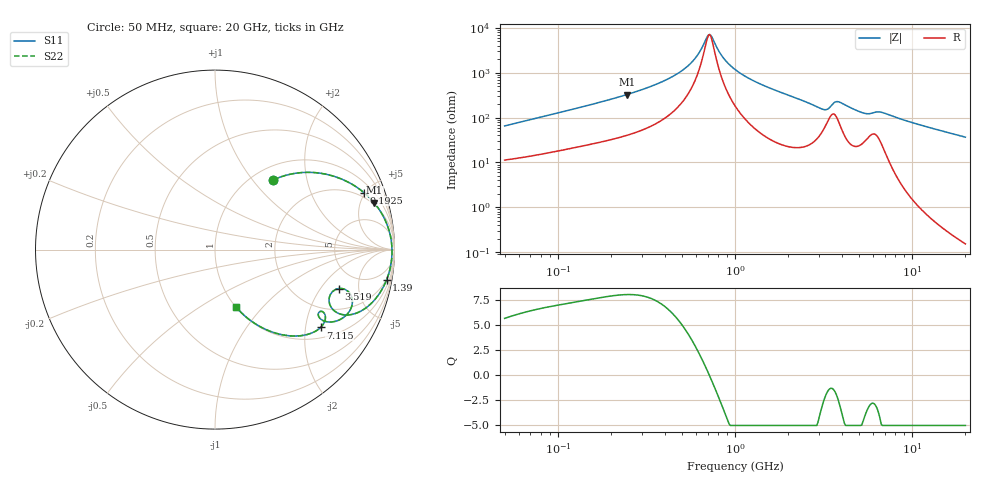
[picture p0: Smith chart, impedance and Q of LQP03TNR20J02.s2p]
!Murata Part Number: LQP03TNR20J02
!These Parameters are Measured in Series Mode Connection
!  o--[Z]--o
!Port1  Port2
!  o-------o
!Freq. Start=50[MHz] Stop=20[GHz], 401[Steps]
# Hz S RI R 50
!Freq.(Hz) S11(Real) S11(Imag) S21(Real) S21(Imag) S12(Real) S12(Imag) S22(Real) S22(Imag)
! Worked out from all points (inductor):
!   401 points, 50 MHz to 20 GHz, reference 50 ohm
!   read as one part in series: L = 201 nH near 51.52 MHz
!   highest Q = 8.05 at 244.6 MHz (marker M1), where L = 210 nH
!   self-resonance near 708.6 MHz
!   S11 on the Smith chart (normalised r, x): 50 MHz: 1.23, +1.28; 192.5 MHz: 1.62, +4.90; 1.39 GHz: 2, -11; 3.519 GHz: 3.33, -3.01; 7.115 GHz: 1.30, -2.43; 20 GHz: 1.00, -0.73
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5e7  0.3259 0.3888  0.6741 -0.3888  0.6741 -0.3888  0.3259 0.3888
1.364002e8  0.7228 0.3852  0.2772 -0.3852  0.2772 -0.3852  0.7228 0.3852
1.925012e8  0.8303 0.3171  0.1697 -0.3171  0.1697 -0.3171  0.8303 0.3171
2.446335e8  0.8868 0.2607  0.1132 -0.2607  0.1132 -0.2607  0.8868 0.2607
3.721004e8  0.9514 0.157  0.0486 -0.157  0.0486 -0.157  0.9514 0.157
5.492803e8  0.9799 0.0629  0.0201 -0.0629  0.0201 -0.0629  0.9799 0.0629
6.100003e8  0.9835 0.0381  0.0165 -0.0381  0.0165 -0.0381  0.9835 0.0381
7.192613e8  0.9862 -0.000867  0.0138 0.000867  0.0138 0.000867  0.9862 -0.000867
8.608917e8  0.9849 -0.0439  0.0151 0.0439  0.0151 0.0439  0.9849 -0.0439
1e9  0.9804 -0.0808  0.0196 0.0808  0.0196 0.0808  0.9804 -0.0808
1.390315e9  0.9564 -0.1677  0.0436 0.1677  0.0436 0.1677  0.9564 -0.1677
2.728004e9  0.7625 -0.3613  0.2375 0.3613  0.2375 0.3613  0.7625 -0.3613
3.216634e9  0.6392 -0.3053  0.3608 0.3053  0.3608 0.3053  0.6392 -0.3053
3.519108e9  0.6888 -0.2169  0.3112 0.2169  0.3112 0.2169  0.6888 -0.2169
3.967106e9  0.7646 -0.3033  0.2354 0.3033  0.2354 0.3033  0.7646 -0.3033
4.677679e9  0.6794 -0.3969  0.3206 0.3969  0.3206 0.3969  0.6794 -0.3969
5.515528e9  0.5794 -0.3758  0.4206 0.3758  0.4206 0.3758  0.5794 -0.3758
6.125241e9  0.5982 -0.3454  0.4018 0.3454  0.4018 0.3454  0.5982 -0.3454
7.114996e9  0.5884 -0.4335  0.4116 0.4335  0.4116 0.4335  0.5884 -0.4335
7.442007e9  0.5618 -0.4537  0.4382 0.4537  0.4382 0.4537  0.5618 -0.4537
1.220001e10  0.2786 -0.4429  0.7214 0.4429  0.7214 0.4429  0.2786 -0.4429
2e10  0.1196 -0.3224  0.8804 0.3224  0.8804 0.3224  0.1196 -0.3224
